| This Model is valid for Industrial grade Temperature Range -40C<=Tc<=95C
| Valid for DDR3/DDR3L-1866/2133 operation
| Part Number   VDDQ   Package   Architecture
| SCB13H1G160EF   1.35 +0.1/-0.067   BGA   1G bit x 16
| SCB15H1G160EF   1.5  +0.075/-0.075   BGA   1G bit x 16
[IBIS ver] 5.0
[File name]  ussxh1g16ei.ibs
[File Rev]  1.0
[Date]   November 6, 2023
[Source] Simulation of a silicon level SPICE model
[Notes]  IBIS Characteristics for I/O Buffer
  IBIS Model Revision History: Rev 1.0:
  2023-11-06 - IBIS model file initial creation
[Disclaimer]  The IBIS models are for modeling purpose only and are subject to change without any notice. UniIC is not
  responsible for any problems the models may cause.
[Copyright] Copyright 2023 UniIC Semiconductors Corp. All rights reserved
|   Component SCB13H1G160EF
[Component] SCB13H1G160EF
[Manufacturer] UniIC Semiconductors Corp.
[Package]
| variable   typ   min   max
R_pkg   1.000   0.835   1.170
L_pkg   3.360nH   2.810nH   3.910nH
C_pkg   0.624pF   0.488pF   0.760pF
[Pin]  signal_name   model_name   R_pin   L_pin   C_pin
A1   VDDQ   Power
A2   DQU5   DQ   1.170   3.910nH   0.760pF
A3   DQU7   DQ   1.120   3.790nH   0.723pF
A7   DQU4   DQ   1.080   3.510nH   0.687pF
A8   VDDQ   Power
A9   VSS   Gnd
B1   VSS   Gnd
B2   VDD   Power
B3   VSS   Gnd
B7   DQSU#   DQ   0.990   3.380nH   0.697pF
B8   DQU6   DQ   0.874   2.920nH   0.557pF
B9   VSS   Gnd
C1   VDDQ   Power
C2   DQU3   DQ   0.860   3.360nH   0.586pF
C3   DQU1   DQ   1.020   3.570nH   0.683pF
C7   DQSU   DQ   0.959   3.380nH   0.680pF
C8   DQU2   DQ   0.869   3.200nH   0.614pF
C9   VDDQ   Power
D1   VSS   Gnd
D2   VDDQ   Power
D3   DMU   DQ   0.855   3.340nH   0.548pF
D7   DQU0   DQ   0.892   3.570nH   0.630pF
D8   VSS   Gnd
D9   VDD   Power
E1   VSS   Gnd
E2   VSS   Gnd
E3   DQL0   DQ   0.836   3.120nH   0.531pF
E7   DML   DQ   0.861   3.130nH   0.551pF
E8   VSS   Gnd
E9   VDDQ   Power
F1   VDDQ   Power
F2   DQL2   DQ   0.818   3.130nH   0.544pF
F3   DQSL   DQ   0.805   2.900nH   0.493pF
F7   DQL1   DQ   0.813   2.970nH   0.527pF
F8   DQL3   DQ   0.942   3.080nH   0.661pF
F9   VSS   Gnd
G1   VSS   Gnd
G2   DQL6   DQ   0.875   2.920nH   0.557pF
G3   DQSL#   DQ   0.835   2.820nH   0.488pF
G7   VDD   Power
G8   VSS   Gnd
G9   VSS   Gnd
H1   VREFDQ   Power
H2   VDDQ   Power
H3   DQL4   DQ   0.760   2.730nH   0.437pF
H7   DQL7   DQ   0.858   3.390nH   0.596pF
H8   DQL5   DQ   0.811   3.040nH   0.476pF
H9   VDDQ   Power
J1   NC1   NC
J2   VSS   Gnd
J3   RAS#   CA   0.327   1.220nH   0.290pF
J7   CK   CA   0.751   2.470nH   0.463pF
J8   VSS   Gnd
J9   NC2   NC
K1   ODT   RCV_ODT   0.712   2.600nH   0.513pF
K2   VDD   Power
K3   CAS#   CA   0.683   2.640nH   0.434pF
K7   CK#   CA   0.759   2.580nH   0.438pF
K8   VDD   Power
K9   CKE   CA   0.731   2.760nH   0.535pF
L1   NC3   NC
L2   CS#   CA   0.739   2.750nH   0.509pF
L3   WE#   CA   0.461   1.860nH   0.376pF
L7   A10   CA   0.738   2.790nH   0.436pF
L8   ZQ   Power
L9   NC4   NC
M1   VSS   Gnd
M2   BA0   CA   0.787   2.860nH   0.532pF
M3   BA2   CA   0.798   2.610nH   0.582pF
M7   NC5   NC
M8   VREFCA   Power
M9   VSS   Gnd
N1   VDD   Power
N2   A3   CA   0.858   2.810nH   0.595pF
N3   A0   CA   0.760   3.030nH   0.518pF
N7   A12   CA   0.734   2.840nH   0.536pF
N8   BA1   CA   0.737   3.030nH   0.523pF
N9   VDD   Power
P1   VSS   Gnd
P2   A5   CA   0.784   3.250nH   0.583pF
P3   A2   CA   0.651   2.880nH   0.509pF
P7   A1   CA   0.698   3.010nH   0.509pF
P8   A4   CA   0.814   3.150nH   0.602pF
P9   VSS   Gnd
R1   VDD   Power
R2   A7   CA   0.861   3.550nH   0.599pF
R3   A9   CA   0.802   4.220nH   0.682pF
R7   A11   CA   0.856   3.390nH   0.600pF
R8   A6   CA   0.896   3.830nH   0.611pF
R9   VDD   Power
T1   VSS   Gnd
T2   RESET#   RST_N
T3   NC6   NC
T7   NC7   NC
T8   A8   CA   1.020   4.220nH   0.682pF
T9   VSS   Gnd
|IN   dq_in   dummy
|EN   dq_en   dummy
[Diff pin]  inv_pin  vdiff   tdelay_typ   tdelay_min   tdelay_max
C7   B7   0.270V   NA   NA   NA
F3   G3   0.270V   NA   NA   NA
J7   K7   0.270V   NA   NA   NA
|   Component SCB15H1G160EF
[Component] SCB15H1G160EF
[Manufacturer] UniIC Semiconductors Corp.
[Package]
| variable   typ   min   max
R_pkg   1.000   0.835   1.170
L_pkg   3.360nH   2.810nH   3.910nH
C_pkg   0.624pF   0.488pF   0.760pF
[Pin]  signal_name   model_name   R_pin   L_pin   C_pin
A1   VDDQ   Power
A2   DQU5   DQ   1.170   3.910nH   0.760pF
A3   DQU7   DQ   1.120   3.790nH   0.723pF
A7   DQU4   DQ   1.080   3.510nH   0.687pF
A8   VDDQ   Power
A9   VSS   Gnd
B1   VSS   Gnd
B2   VDD   Power
B3   VSS   Gnd
B7   DQSU#   DQ   0.990   3.380nH   0.697pF
B8   DQU6   DQ   0.874   2.920nH   0.557pF
B9   VSS   Gnd
C1   VDDQ   Power
C2   DQU3   DQ   0.860   3.360nH   0.586pF
C3   DQU1   DQ   1.020   3.570nH   0.683pF
C7   DQSU   DQ   0.959   3.380nH   0.680pF
C8   DQU2   DQ   0.869   3.200nH   0.614pF
C9   VDDQ   Power
D1   VSS   Gnd
D2   VDDQ   Power
D3   DMU   DQ   0.855   3.340nH   0.548pF
D7   DQU0   DQ   0.892   3.570nH   0.630pF
D8   VSS   Gnd
D9   VDD   Power
E1   VSS   Gnd
E2   VSS   Gnd
E3   DQL0   DQ   0.836   3.120nH   0.531pF
E7   DML   DQ   0.861   3.130nH   0.551pF
E8   VSS   Gnd
E9   VDDQ   Power
F1   VDDQ   Power
F2   DQL2   DQ   0.818   3.130nH   0.544pF
F3   DQSL   DQ   0.805   2.900nH   0.493pF
F7   DQL1   DQ   0.813   2.970nH   0.527pF
F8   DQL3   DQ   0.942   3.080nH   0.661pF
F9   VSS   Gnd
G1   VSS   Gnd
G2   DQL6   DQ   0.875   2.920nH   0.557pF
G3   DQSL#   DQ   0.835   2.820nH   0.488pF
G7   VDD   Power
G8   VSS   Gnd
G9   VSS   Gnd
H1   VREFDQ   Power
H2   VDDQ   Power
H3   DQL4   DQ   0.760   2.730nH   0.437pF
H7   DQL7   DQ   0.858   3.390nH   0.596pF
H8   DQL5   DQ   0.811   3.040nH   0.476pF
H9   VDDQ   Power
J1   NC1   NC
J2   VSS   Gnd
J3   RAS#   CA   0.327   1.220nH   0.290pF
J7   CK   CA   0.751   2.470nH   0.463pF
J8   VSS   Gnd
J9   NC2   NC
K1   ODT   RCV_ODT   0.712   2.600nH   0.513pF
K2   VDD   Power
K3   CAS#   CA   0.683   2.640nH   0.434pF
K7   CK#   CA   0.759   2.580nH   0.438pF
K8   VDD   Power
K9   CKE   CA   0.731   2.760nH   0.535pF
L1   NC3   NC
L2   CS#   CA   0.739   2.750nH   0.509pF
L3   WE#   CA   0.461   1.860nH   0.376pF
L7   A10   CA   0.738   2.790nH   0.436pF
L8   ZQ   Power
L9   NC4   NC
M1   VSS   Gnd
M2   BA0   CA   0.787   2.860nH   0.532pF
M3   BA2   CA   0.798   2.610nH   0.582pF
M7   NC5   NC
M8   VREFCA   Power
M9   VSS   Gnd
N1   VDD   Power
N2   A3   CA   0.858   2.810nH   0.595pF
N3   A0   CA   0.760   3.030nH   0.518pF
N7   A12   CA   0.734   2.840nH   0.536pF
N8   BA1   CA   0.737   3.030nH   0.523pF
N9   VDD   Power
P1   VSS   Gnd
P2   A5   CA   0.784   3.250nH   0.583pF
P3   A2   CA   0.651   2.880nH   0.509pF
P7   A1   CA   0.698   3.010nH   0.509pF
P8   A4   CA   0.814   3.150nH   0.602pF
P9   VSS   Gnd
R1   VDD   Power
R2   A7   CA   0.861   3.550nH   0.599pF
R3   A9   CA   0.802   4.220nH   0.682pF
R7   A11   CA   0.856   3.390nH   0.600pF
R8   A6   CA   0.896   3.830nH   0.611pF
R9   VDD   Power
T1   VSS   Gnd
T2   RESET#   RST_N
T3   NC6   NC
T7   NC7   NC
T8   A8   CA   1.020   4.220nH   0.682pF
T9   VSS   Gnd
[Diff pin]  inv_pin  vdiff   tdelay_typ   tdelay_min   tdelay_max
C7   B7   0.270V   NA   NA   NA
F3   G3   0.270V   NA   NA   NA
J7   K7   0.270V   NA   NA   NA
[Model Selector] DQ
DQ_RON60_DDR3  DQ/ DQS RON=60ohms, for DDR3
DQ_RON60_DDR3L  DQ/ DQS RON=60ohms, for DDR3L
DQ_RON48_DDR3  DQ/ DQS RON=48ohms, for DDR3
DQ_RON48_DDR3L  DQ/ DQS RON=48ohms, for DDR3L
DQ_RON40_DDR3  DQ/ DQS RON=40ohms, for DDR3
DQ_RON40_DDR3L  DQ/ DQS RON=40ohms, for DDR3L
DQ_RON34_DDR3  DQ/ DQS RON=34ohms, for DDR3
DQ_RON34_DDR3L  DQ/ DQS RON=34ohms, for DDR3L
DQ_RCV_ODTOFF_DDR3  DQ/DM RCV ODTOFF, for DDR3
DQ_RCV_ODTOFF_DDR3L  DQ/DM RCV ODTOFF, for DDR3L
DQ_RCV_ODT120_DDR3  DQ/DM RCV ODT120, for DDR3
DQ_RCV_ODT120_DDR3L  DQ/DM RCV ODT120, for DDR3L
DQ_RCV_ODT60_DDR3  DQ/DM RCV ODT60, for DDR3
DQ_RCV_ODT60_DDR3L  DQ/DM RCV ODT60, for DDR3L
DQ_RCV_ODT40_DDR3  DQ/DM RCV ODT40, for DDR3
DQ_RCV_ODT40_DDR3L  DQ/DM RCV ODT40, for DDR3L
DQ_RCV_ODT30_DDR3  DQ/DM RCV ODT30, for DDR3
DQ_RCV_ODT30_DDR3L  DQ/DM RCV ODT30, for DDR3L
DQ_RCV_ODT20_DDR3  DQ/DM RCV ODT20, for DDR3
DQ_RCV_ODT20_DDR3L  DQ/DM RCV ODT20, for DDR3L
[Model Selector] RST_N
RCV_RST_N_DDR3  RCV RST_N for DDR3
RCV_RST_N_DDR3L  RCV RST_N for DDR3L
[Model Selector] RCV_ODT
RCV_ODT_DDR3  RCV_ODT for DDR3
RCV_ODT_DDR3L  RCV_ODT for DDR3L
[Model Selector] CA
RCV_CA_DDR3  RCV_CA/BA/CS_N/CKE/CKC/CKT/CAS_N/RAS_N/WE_N for DDR3
RCV_CA_DDR3L  RCV_CA/BA/CS_N/CKE/CKC/CKT/CAS_N/RAS_N/WE_N for DDR3L
| Models and submodels in the file (26): DQ_RON60_DDR3 (I/O), DQ_RON60_DDR3L (I/O), DQ_RON48_DDR3 (I/O), DQ_RON48_DDR3L (I/O), DQ_RON40_DDR3 (I/O), DQ_RON40_DDR3L (I/O), DQ_RON34_DDR3 (I/O), DQ_RON34_DDR3L (I/O), DQ_RCV_ODTOFF_DDR3 (Input), DQ_RCV_ODTOFF_DDR3L (Input), DQ_RCV_ODT120_DDR3 (Input), DQ_RCV_ODT120_DDR3L (Input), DQ_RCV_ODT60_DDR3 (Input), DQ_RCV_ODT60_DDR3L (Input), DQ_RCV_ODT40_DDR3 (Input), DQ_RCV_ODT40_DDR3L (Input), DQ_RCV_ODT30_DDR3 (Input), DQ_RCV_ODT30_DDR3L (Input), DQ_RCV_ODT20_DDR3 (Input), DQ_RCV_ODT20_DDR3L (Input), RCV_CA_DDR3 (Input), RCV_CA_DDR3L (Input), RCV_ODT_DDR3 (Input), RCV_ODT_DDR3L (Input), RCV_RST_N_DDR3 (Input), RCV_RST_N_DDR3L (Input)
